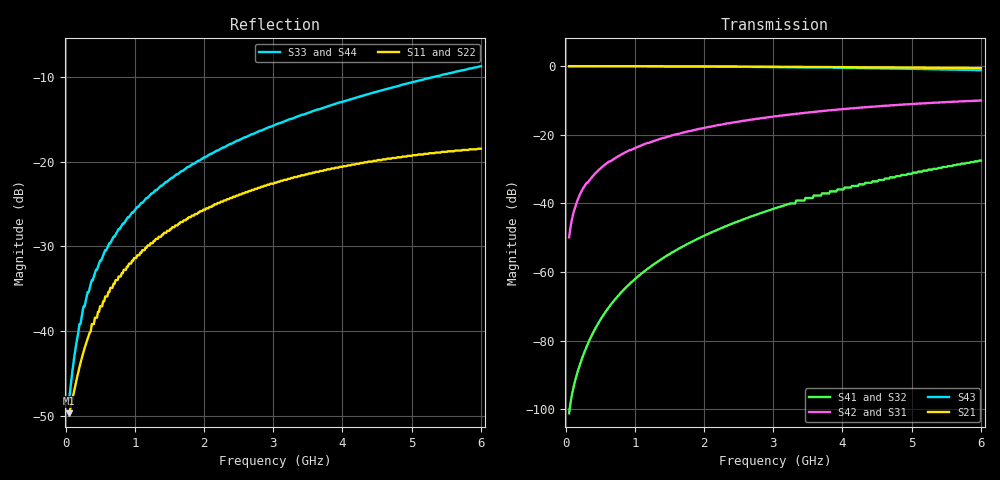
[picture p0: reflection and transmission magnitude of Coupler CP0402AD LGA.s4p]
!	AVX THIN FILM OPERATION
!	CP0402 HIGH DIRECTIVITY COUPLERS
!	P/N CP0402AxxxxDLTR
!	Network	Analyzer HP8720ES.07.64:Feb23,2000 Serial No.US39172382
!	Hewlett-Packard
!	24July2003	02:45:57
# MHZ S MA R 50
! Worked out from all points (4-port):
!   400 points, 50 MHz to 6 GHz, reference 50 ohm
!   strongest paths, dB at 50 MHz, 1.541 GHz, 3.032 GHz, 4.524 GHz, 6 GHz:
!     S21: 0.0, -0.1, -0.2, -0.4, -0.6
!     S43: 0.0, -0.1, -0.3, -0.7, -1.2
!     S42: -49.9, -20.2, -14.6, -11.7, -10.0
!     S31: -49.9, -20.2, -14.6, -11.7, -10.0
!     S41: -101.1, -54.3, -41.4, -33.2, -27.5
!     S32: -101.1, -54.3, -41.4, -33.2, -27.5
!   lowest |S11| = -49.7 dB at 50 MHz (marker M1), VSWR 1.01, Z = 50.3 - j0.137 ohm
!   |S11| at or under -10 dB: start of sweep to end of sweep
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50  0.003276 -24.6  0.997 -0.3  0.003217 89.5  8.782e-06 -92.3
    0.997 -0.3  0.003276 -24.6  8.782e-06 -92.3  0.003217 89.5
    0.003217 89.5  8.782e-06 -92.3  0.003937 40.1  0.997 -0.6
    8.782e-06 -92.3  0.003217 89.5  0.997 -0.6  0.003937 40.1
139.474  0.004789 -52.5  0.997 -1.0  0.008972 88.7  2.679e-05 -114.0
         0.997 -1.0  0.004789 -52.5  2.679e-05 -114.0  0.008972 88.7
         0.008972 88.7  2.679e-05 -114.0  0.007751 65.8  0.997 -1.6
         2.679e-05 -114.0  0.008972 88.7  0.997 -1.6  0.007751 65.8
303.509  0.008675 -72.1  0.997 -2.1  0.02 87.2  8.226e-05 -140.2
         0.997 -2.1  0.008675 -72.1  8.226e-05 -140.2  0.02 87.2
         0.02 87.2  8.226e-05 -140.2  0.016 75.7  0.997 -3.5
         8.226e-05 -140.2  0.02 87.2  0.997 -3.5  0.016 75.7
721.053  0.02 -86.3  0.996 -5.0  0.046 83.4  0.0004089 -164.0
         0.996 -5.0  0.02 -86.3  0.0004089 -164.0  0.046 83.4
         0.046 83.4  0.0004089 -164.0  0.037 77.2  0.995 -8.3
         0.0004089 -164.0  0.046 83.4  0.995 -8.3  0.037 77.2
1183.333  0.032 -92.9  0.994 -8.2  0.076 79.1  0.001115 -173.3
          0.994 -8.2  0.032 -92.9  0.001115 -173.3  0.076 79.1
          0.076 79.1  0.001115 -173.3  0.061 73.8  0.992 -13.5
          0.001115 -173.3  0.076 79.1  0.992 -13.5  0.061 73.8
3330.702  0.081 -110.4  0.973 -22.7  0.202 59.5  0.011 163.6
          0.973 -22.7  0.081 -110.4  0.011 163.6  0.202 59.5
          0.202 59.5  0.011 163.6  0.183 50.8  0.959 -38.2
          0.011 163.6  0.202 59.5  0.959 -38.2  0.183 50.8
6000  0.119 -127.7  0.937 -39.5  0.315 35.6  0.042 130.3
      0.937 -39.5  0.119 -127.7  0.042 130.3  0.315 35.6
      0.315 35.6  0.042 130.3  0.365 20.2  0.872 -69.3
      0.042 130.3  0.315 35.6  0.872 -69.3  0.365 20.2
